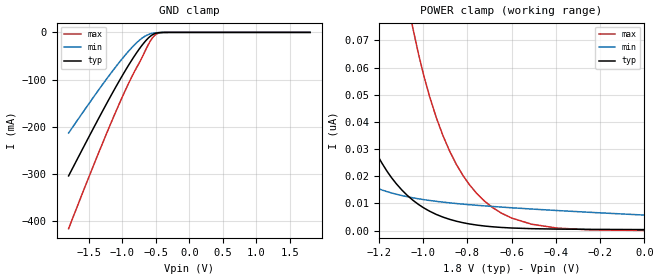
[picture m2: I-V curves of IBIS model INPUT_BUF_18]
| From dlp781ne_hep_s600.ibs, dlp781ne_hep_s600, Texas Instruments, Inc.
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[Model]   INPUT_BUF_18
Model_type  Input
Vinl=0.54
Vinh=1.26
| variable   typ   min   max
C_comp   0.51pF   0.44pF   0.58pF
[Temperature Range]   25   85   -40
[Voltage range]   1.8   1.65   1.95
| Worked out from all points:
|   GND clamp passes 1 mA (typ) near -0.47 V on its own axis
[GND Clamp]
| INPUT_BUF_18
|   Voltage   I(typ)   I(min)   I(max)
-1.8V     -304mA     -213.1mA   -415.8mA
-1.52V    -227.4mA   -155.6mA   -314.4mA
-1.29V    -165.7mA   -109.6mA   -233.4mA
-1.095V   -115.3mA   -72.59mA   -167.6mA
-930mV    -75.06mA   -43.75mA   -115.2mA
-790mV    -43.93mA   -22.51mA   -75.55mA
-680mV    -22.72mA   -9.755mA   -45.56mA
-580mV    -7.998mA   -2.996mA   -17.96mA
-510mV    -2.379mA   -972.8uA   -5.564mA
-450mV    -592.5uA   -304.6uA   -1.296mA
-355mV    -35.15uA   -32.8uA    -61.22uA
1.8V      384pA      6.33nA     42.47pA
[POWER Clamp]
| INPUT_BUF_18
|   Voltage   I(typ)   I(min)   I(max)
-1.8V     438.6nA    109.4nA    1.836uA
-1.7V     293.4nA    73.99nA    1.296uA
-1.565V   164.4nA    44.27nA    784.1nA
-1.4V     75.97nA    25.31nA    401.7nA
-1.255V   36.21nA    17.25nA    210.8nA
-1.155V   20.97nA    14.17nA    130.5nA
-1.045V   11.14nA    12.07nA    74.21nA
-970mV    7.14nA     11.1nA     49.29nA
-880mV    4.163nA    10.23nA    29.33nA
-685mV    1.408nA    8.888nA    8.453nA
-395mV    567.5pA    7.406nA    949.3pA
-16.28fV  384pA      5.724nA    60.79pA
